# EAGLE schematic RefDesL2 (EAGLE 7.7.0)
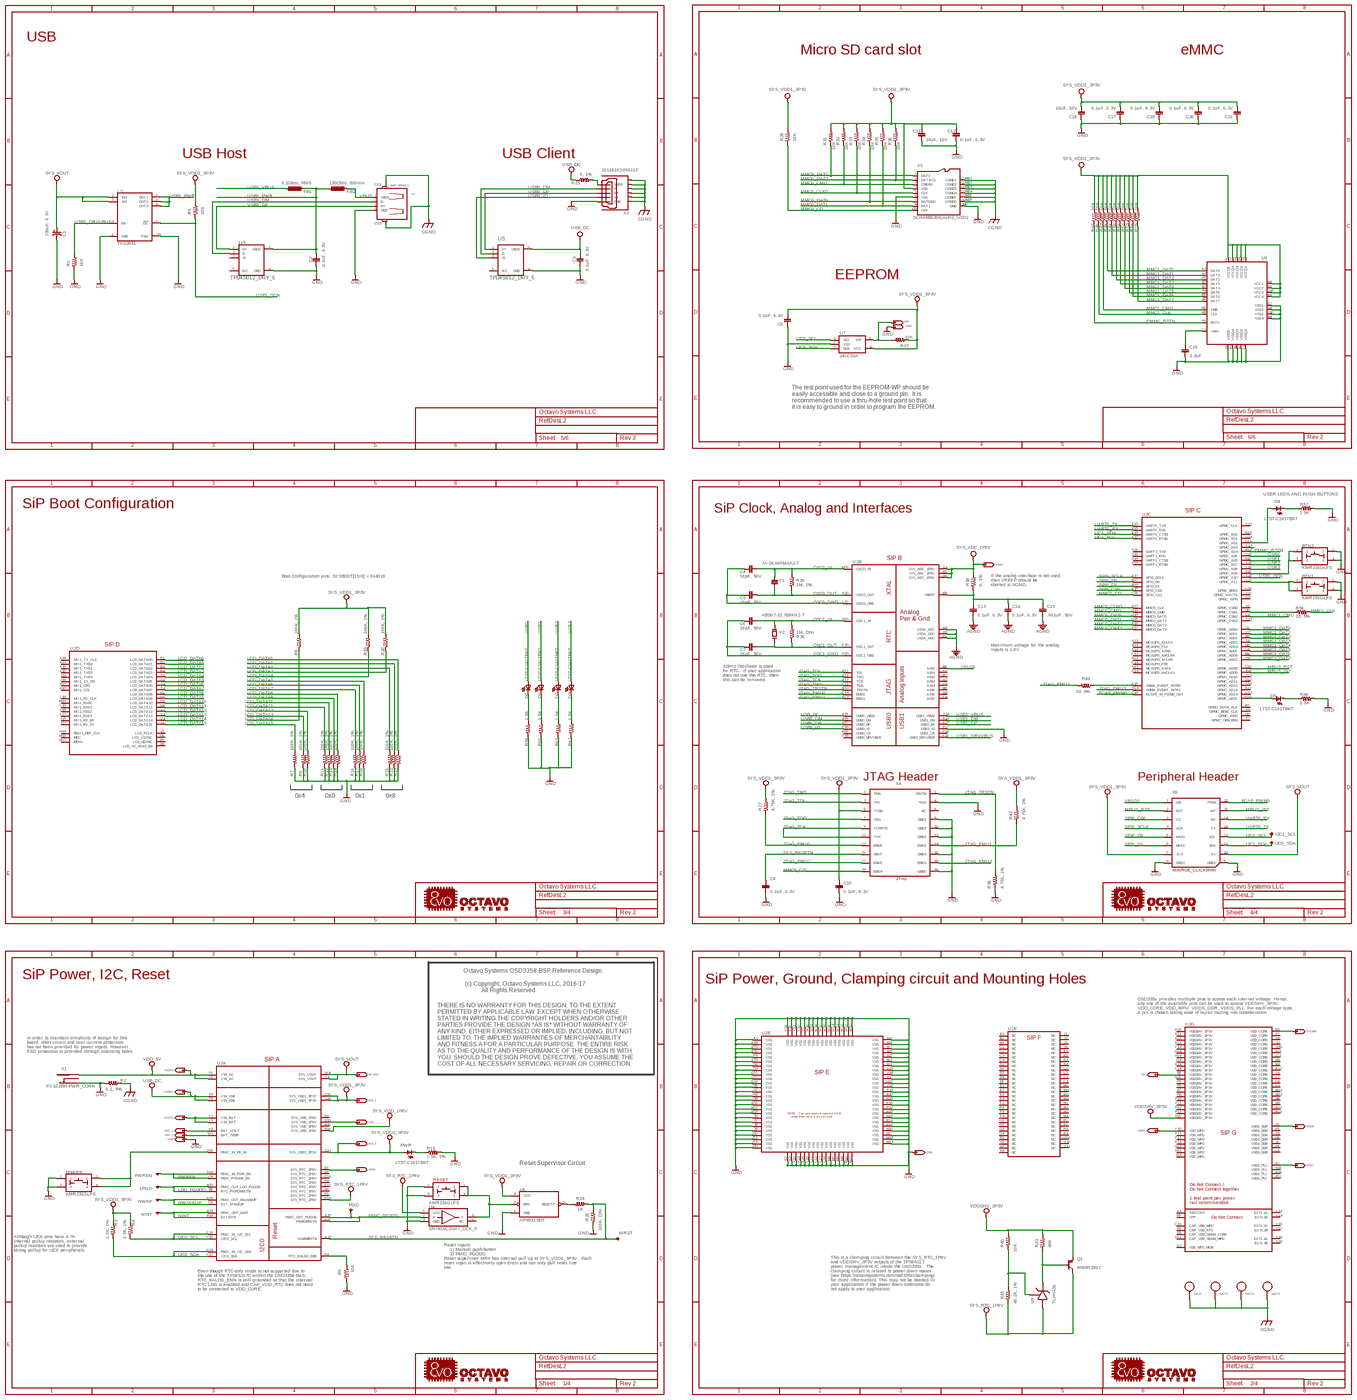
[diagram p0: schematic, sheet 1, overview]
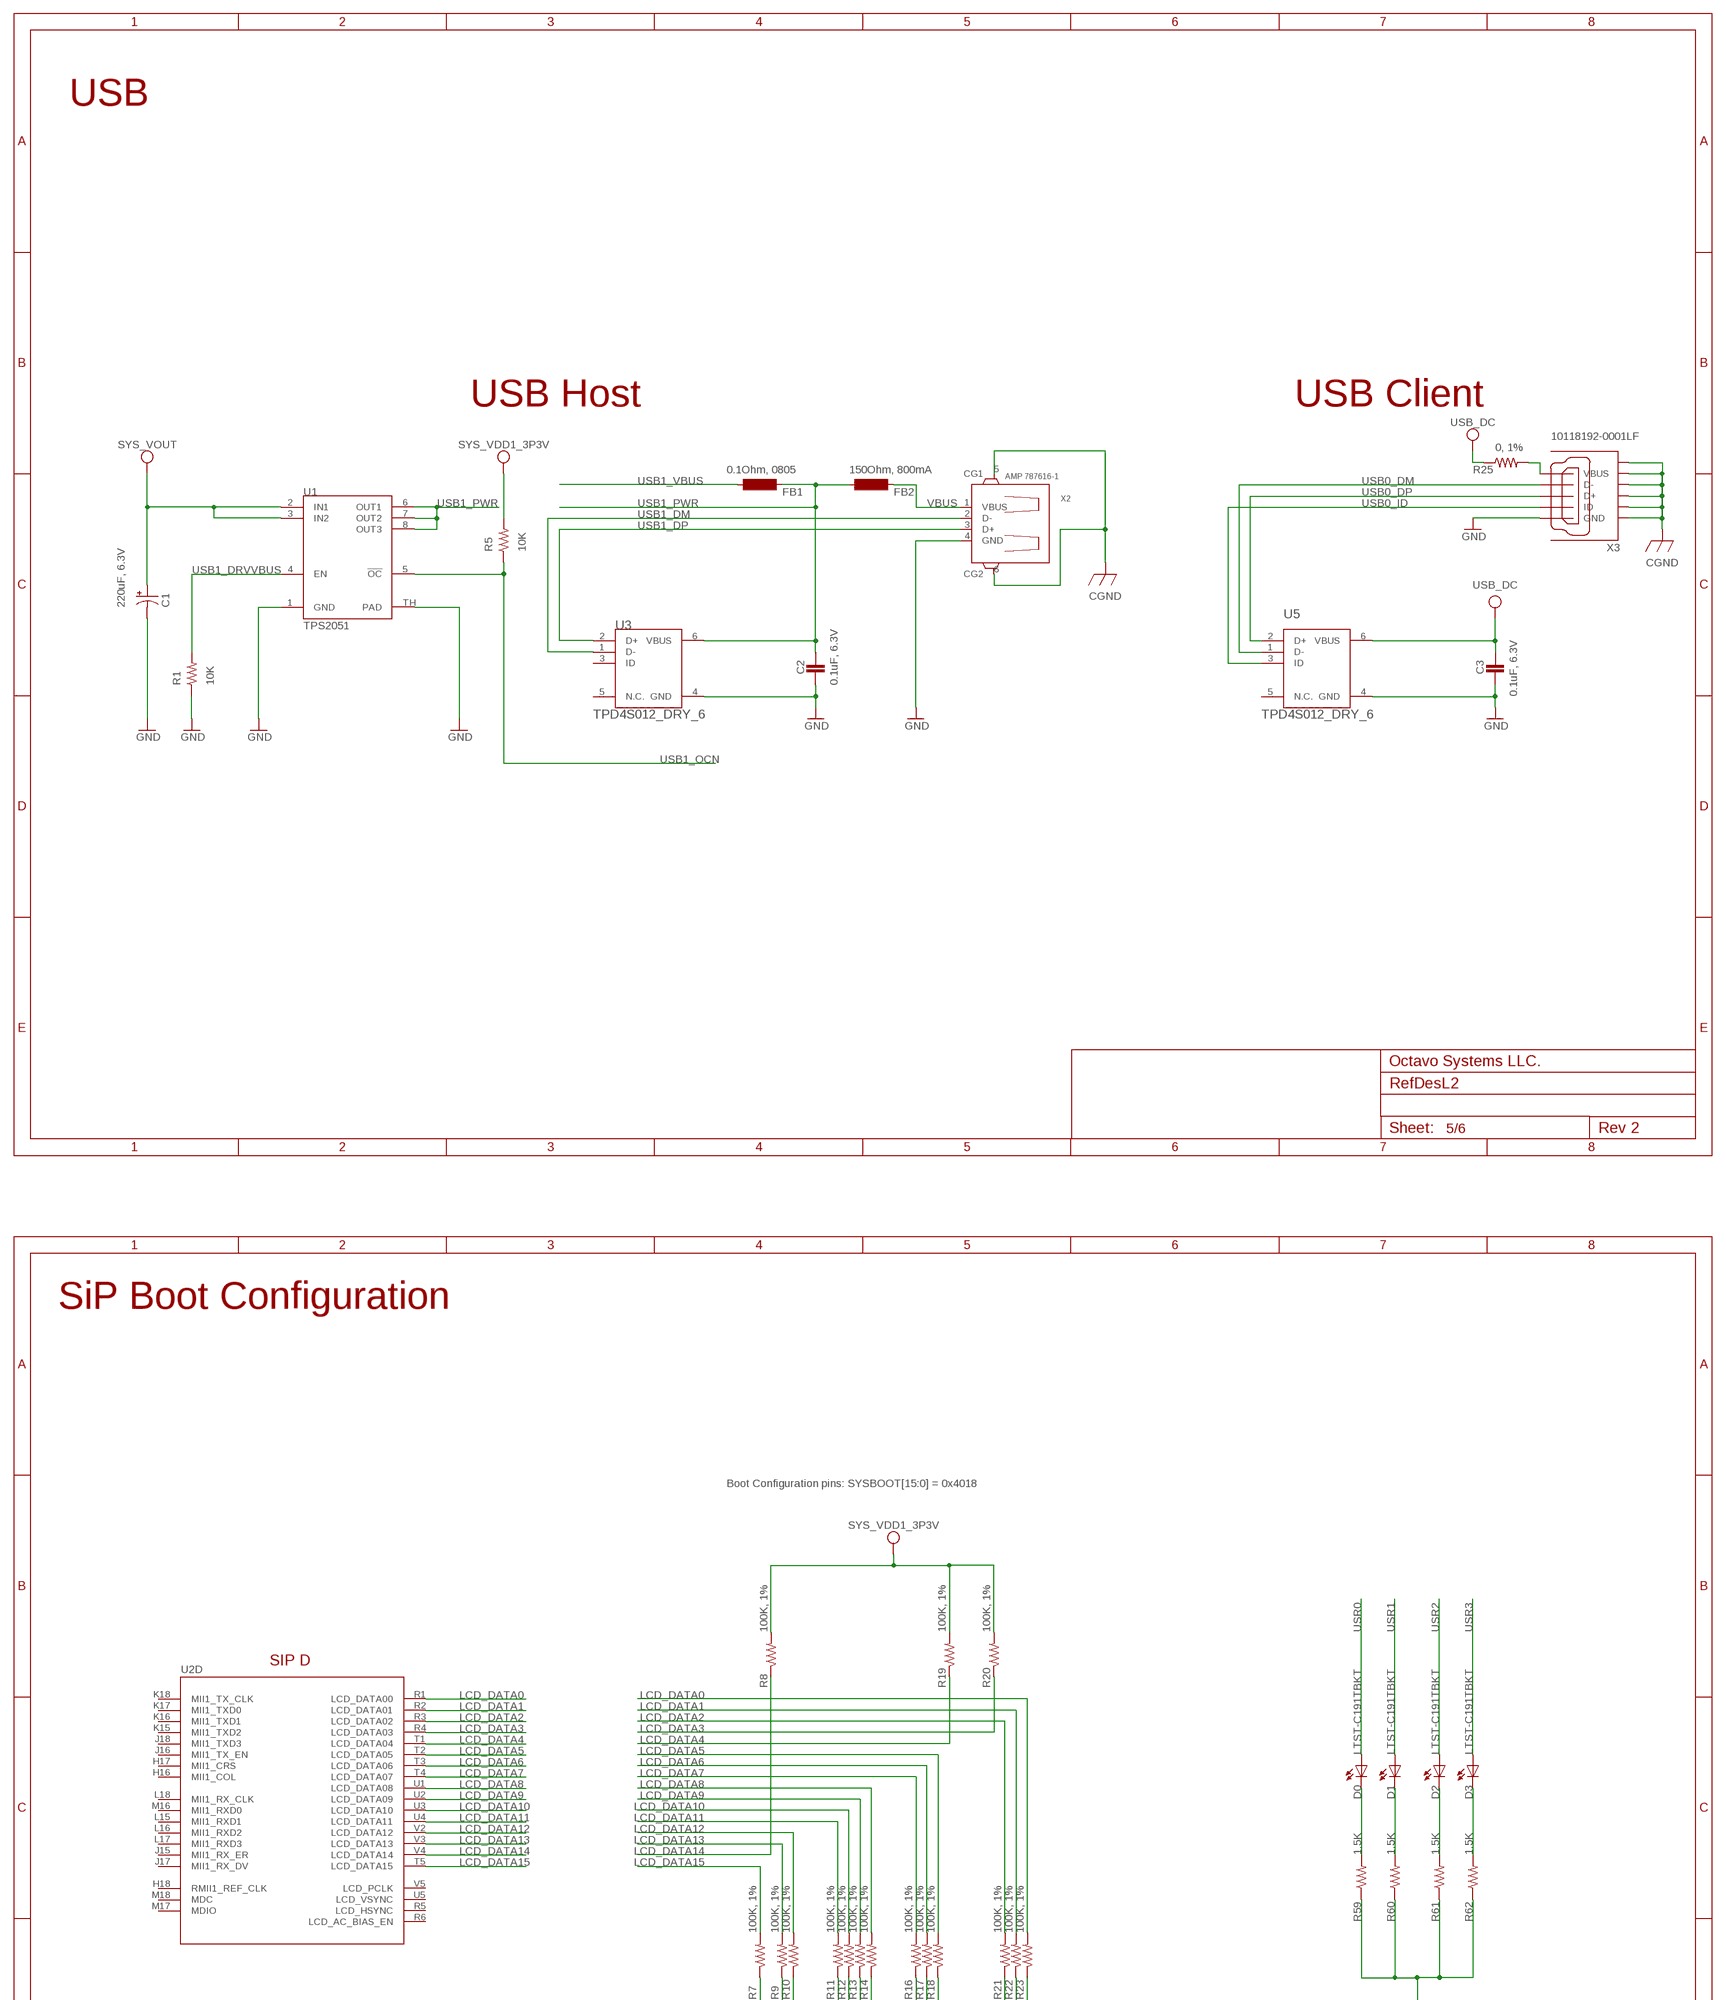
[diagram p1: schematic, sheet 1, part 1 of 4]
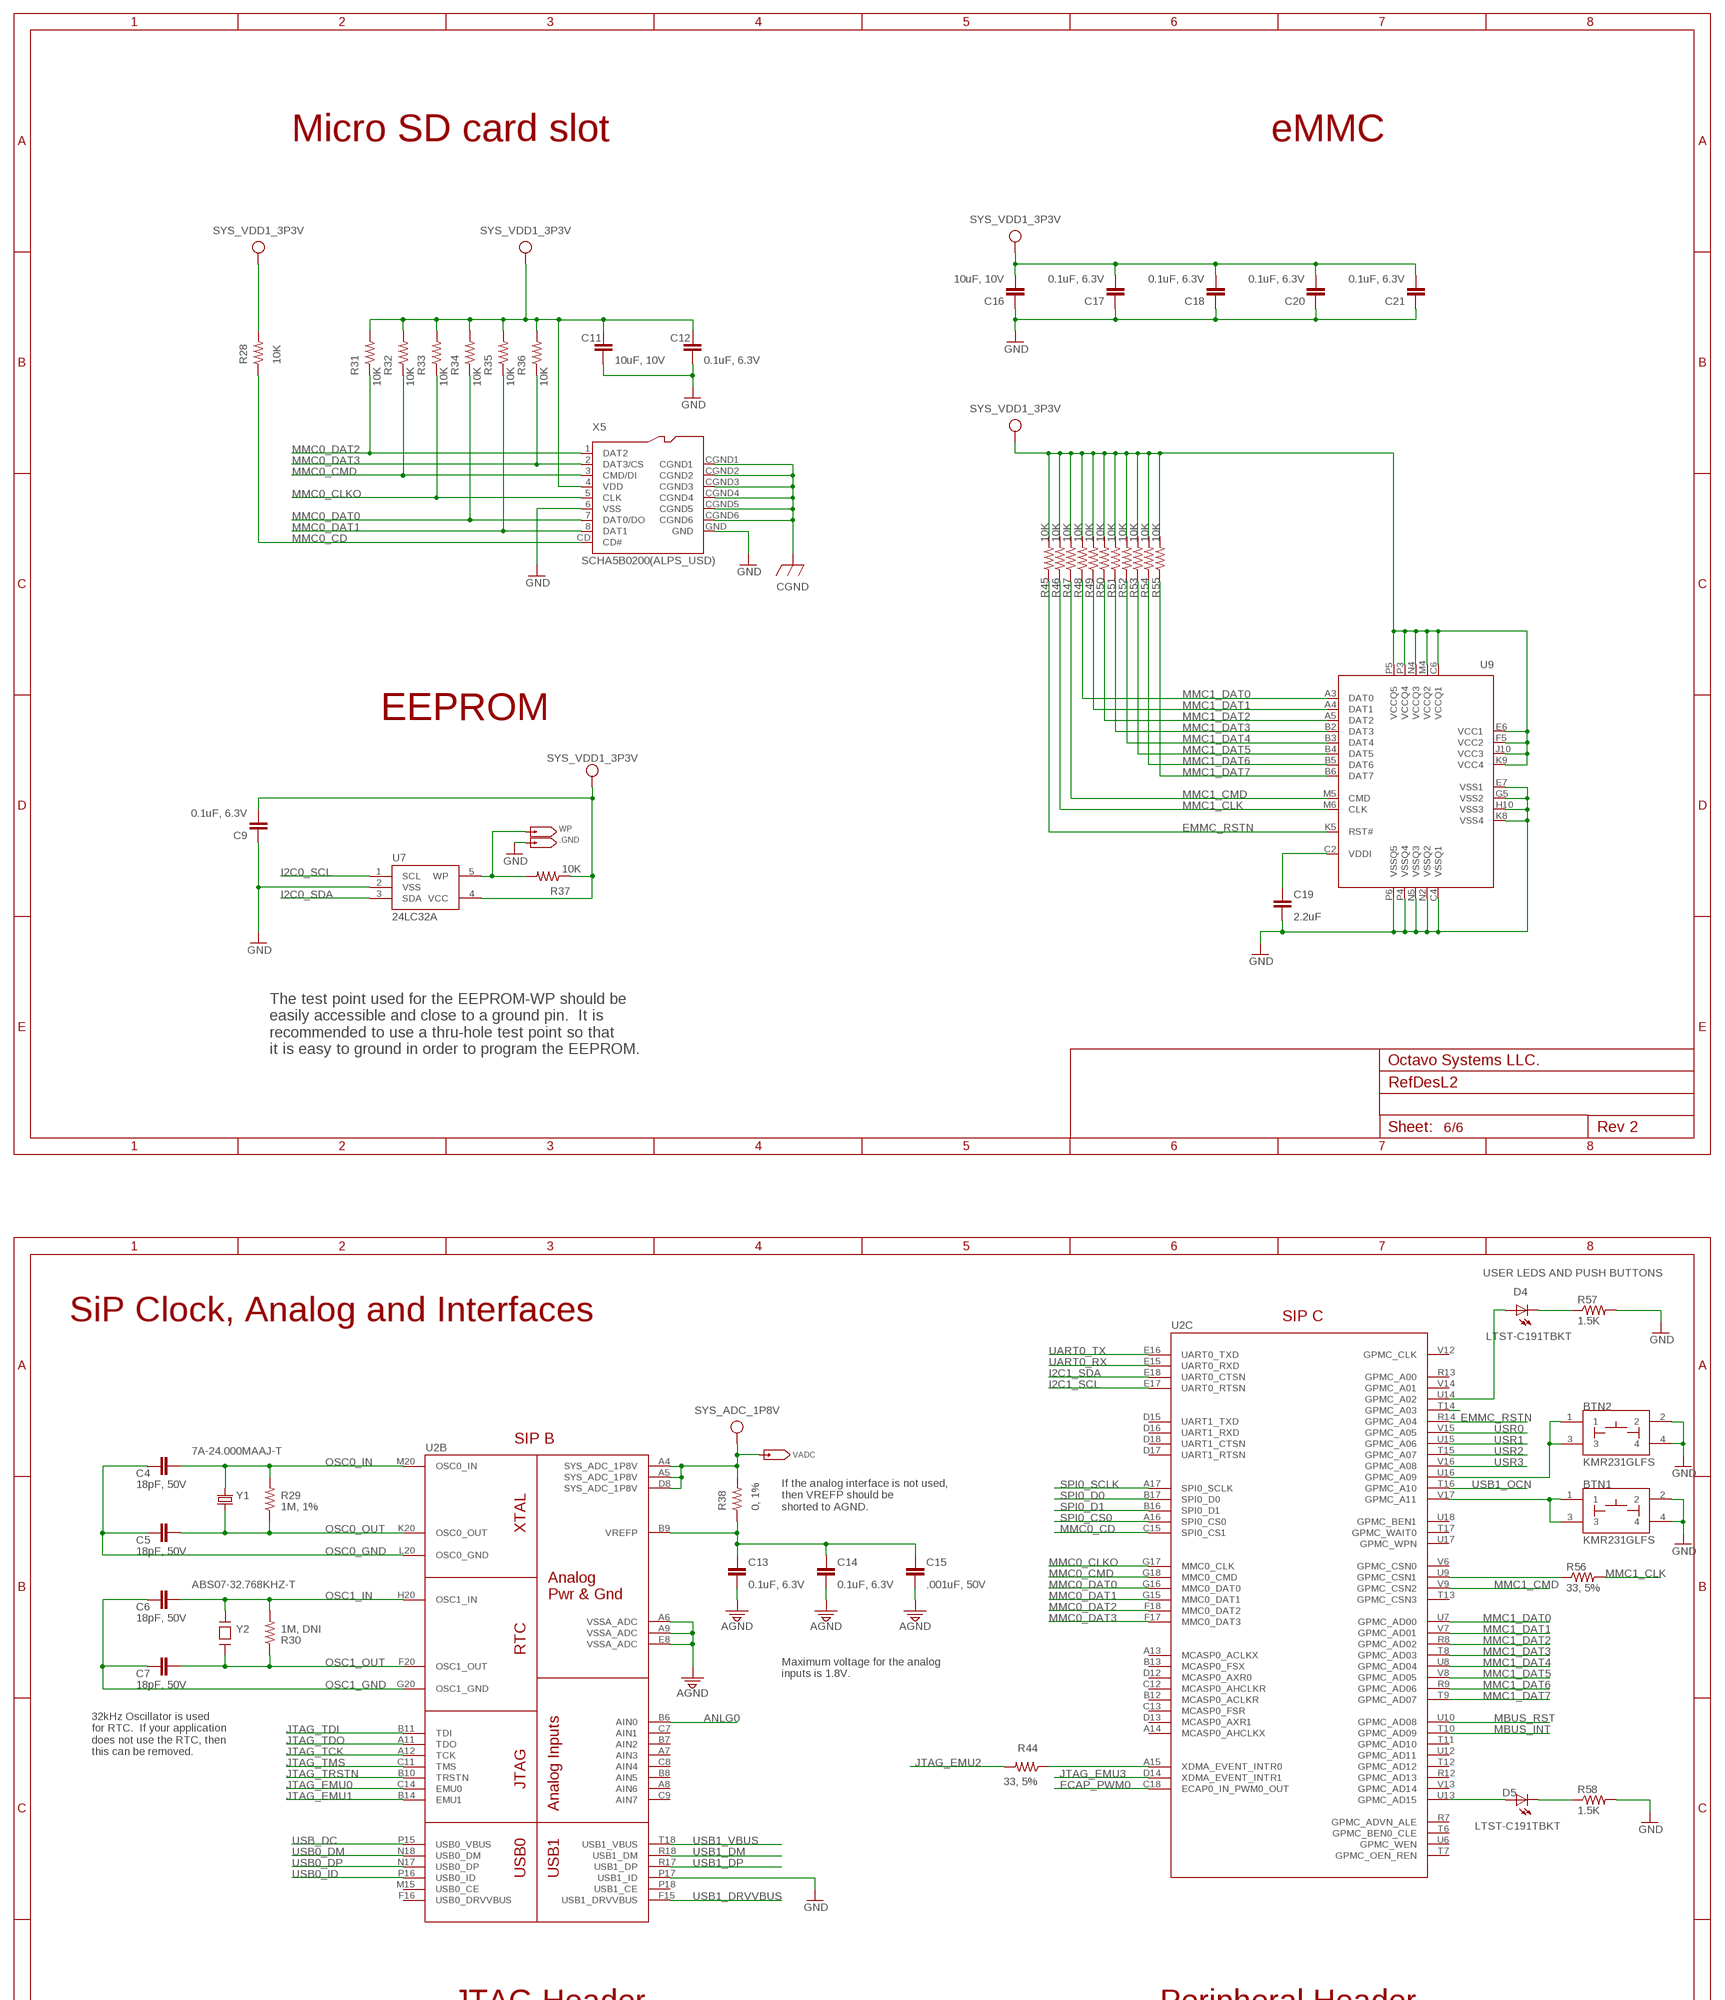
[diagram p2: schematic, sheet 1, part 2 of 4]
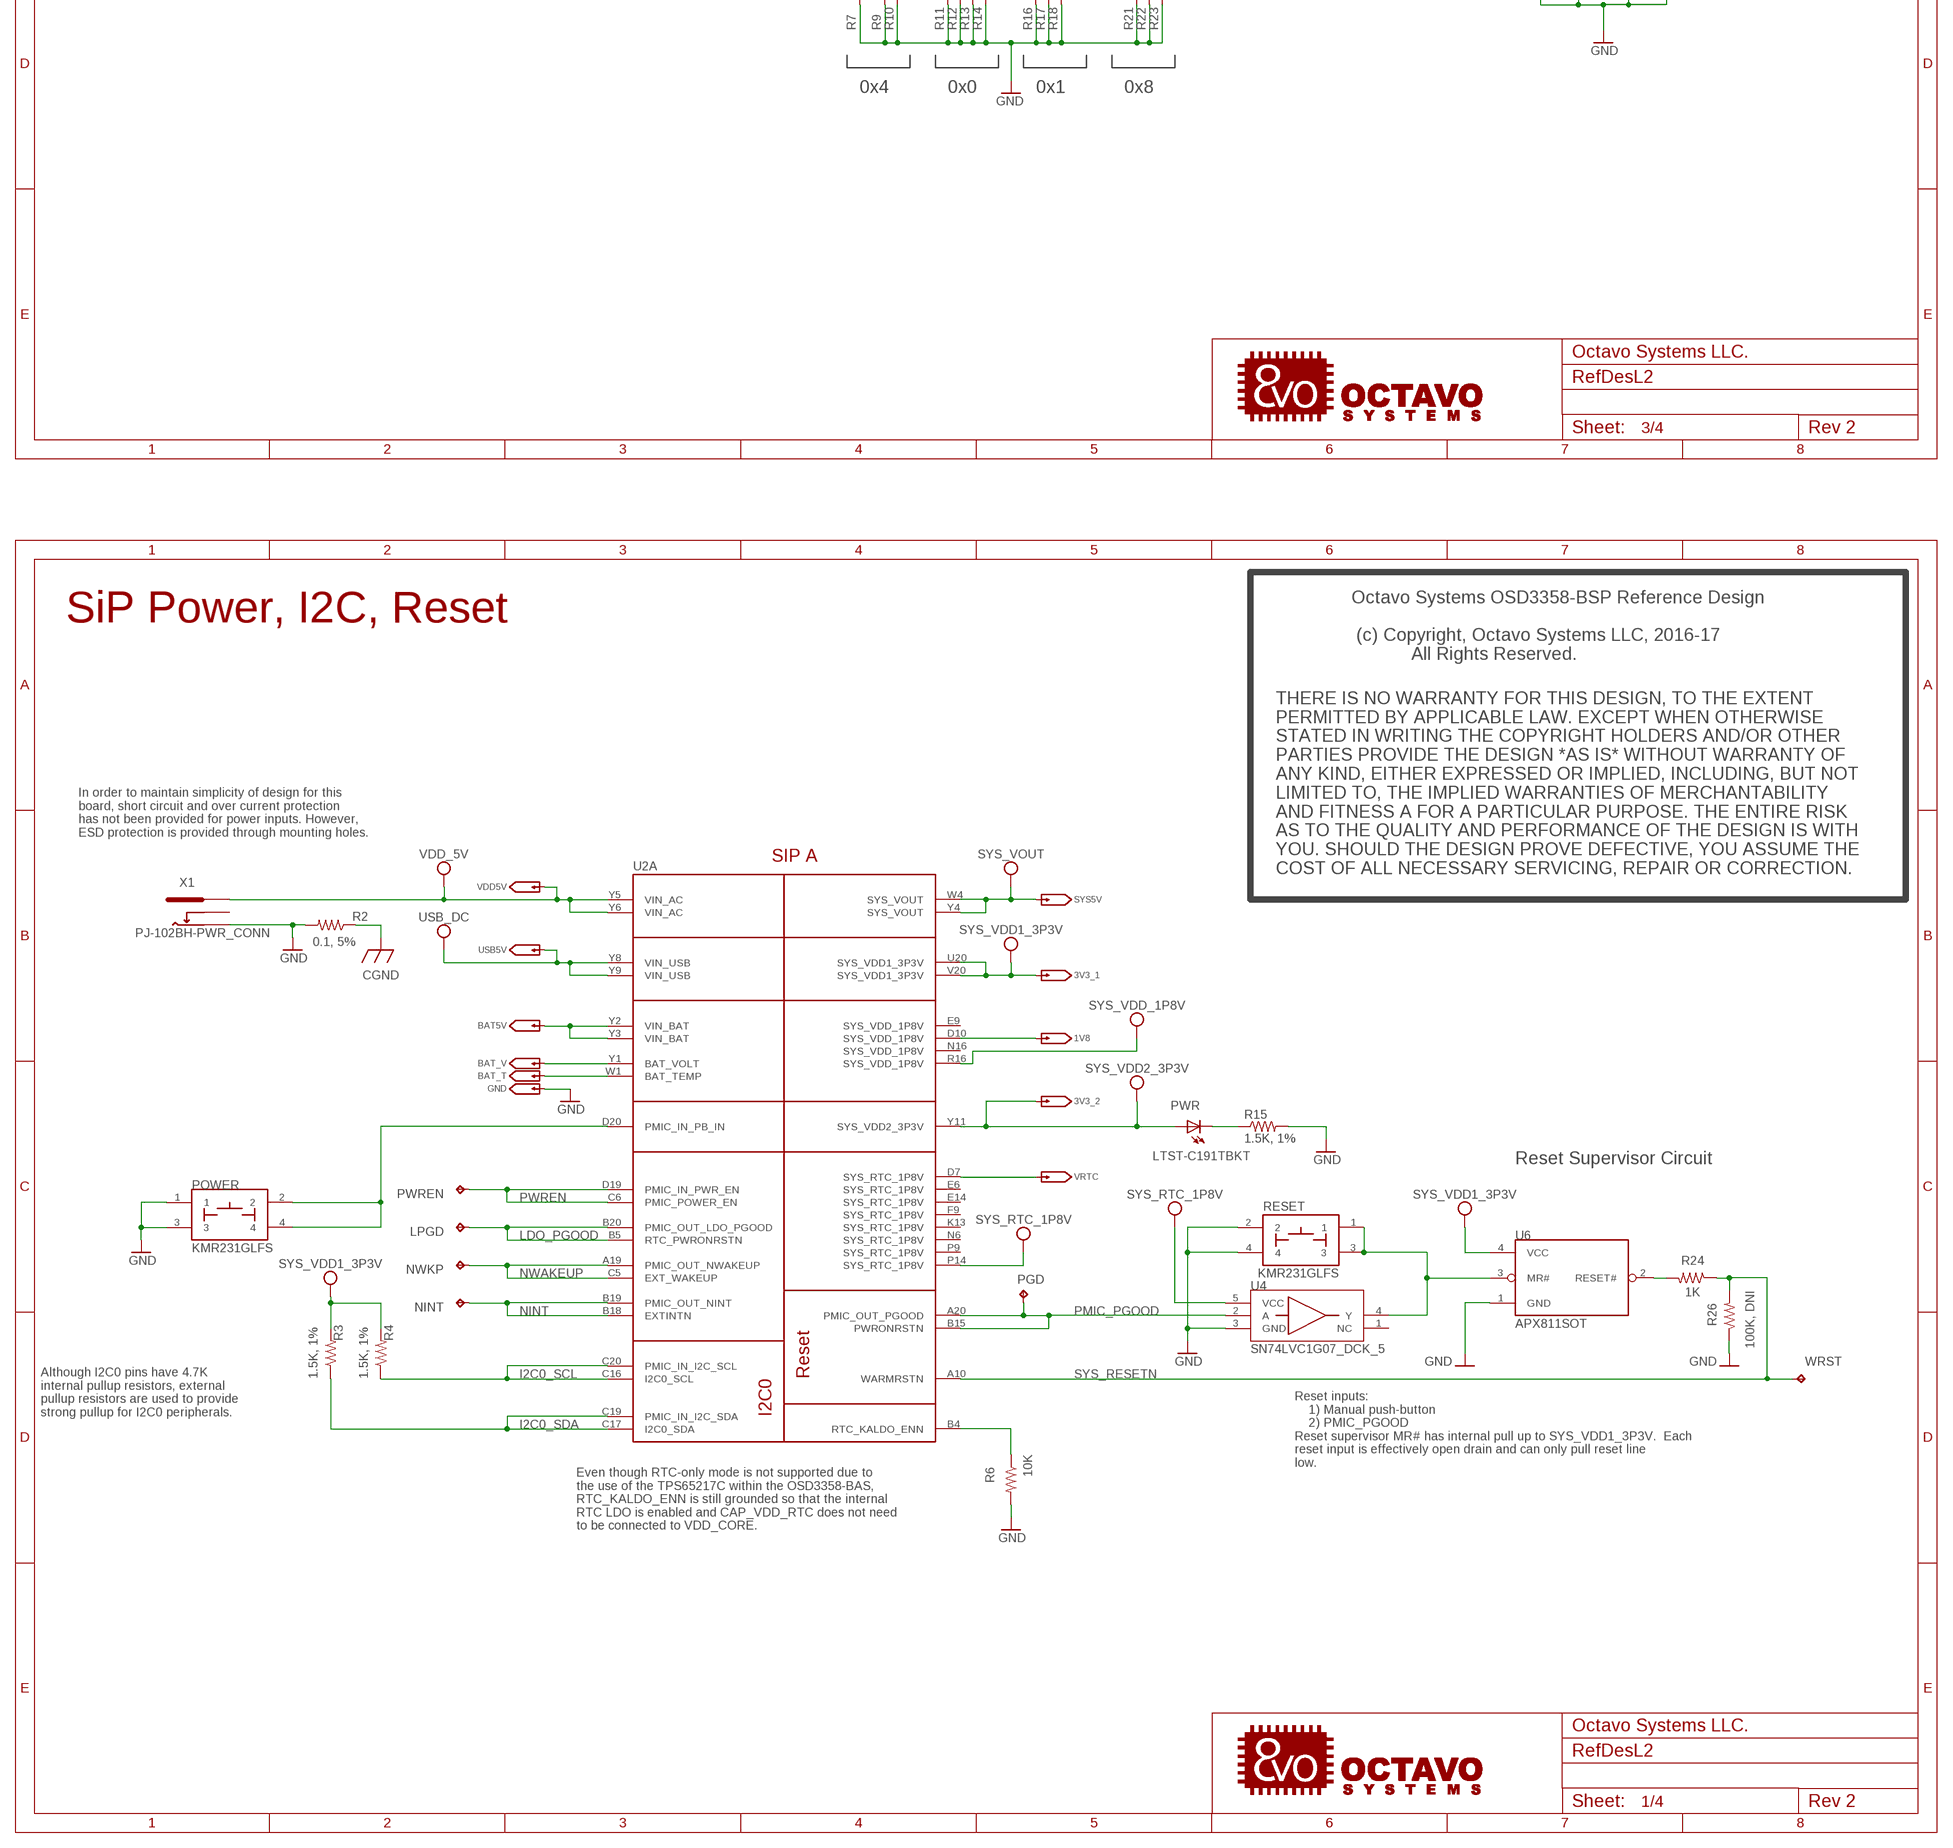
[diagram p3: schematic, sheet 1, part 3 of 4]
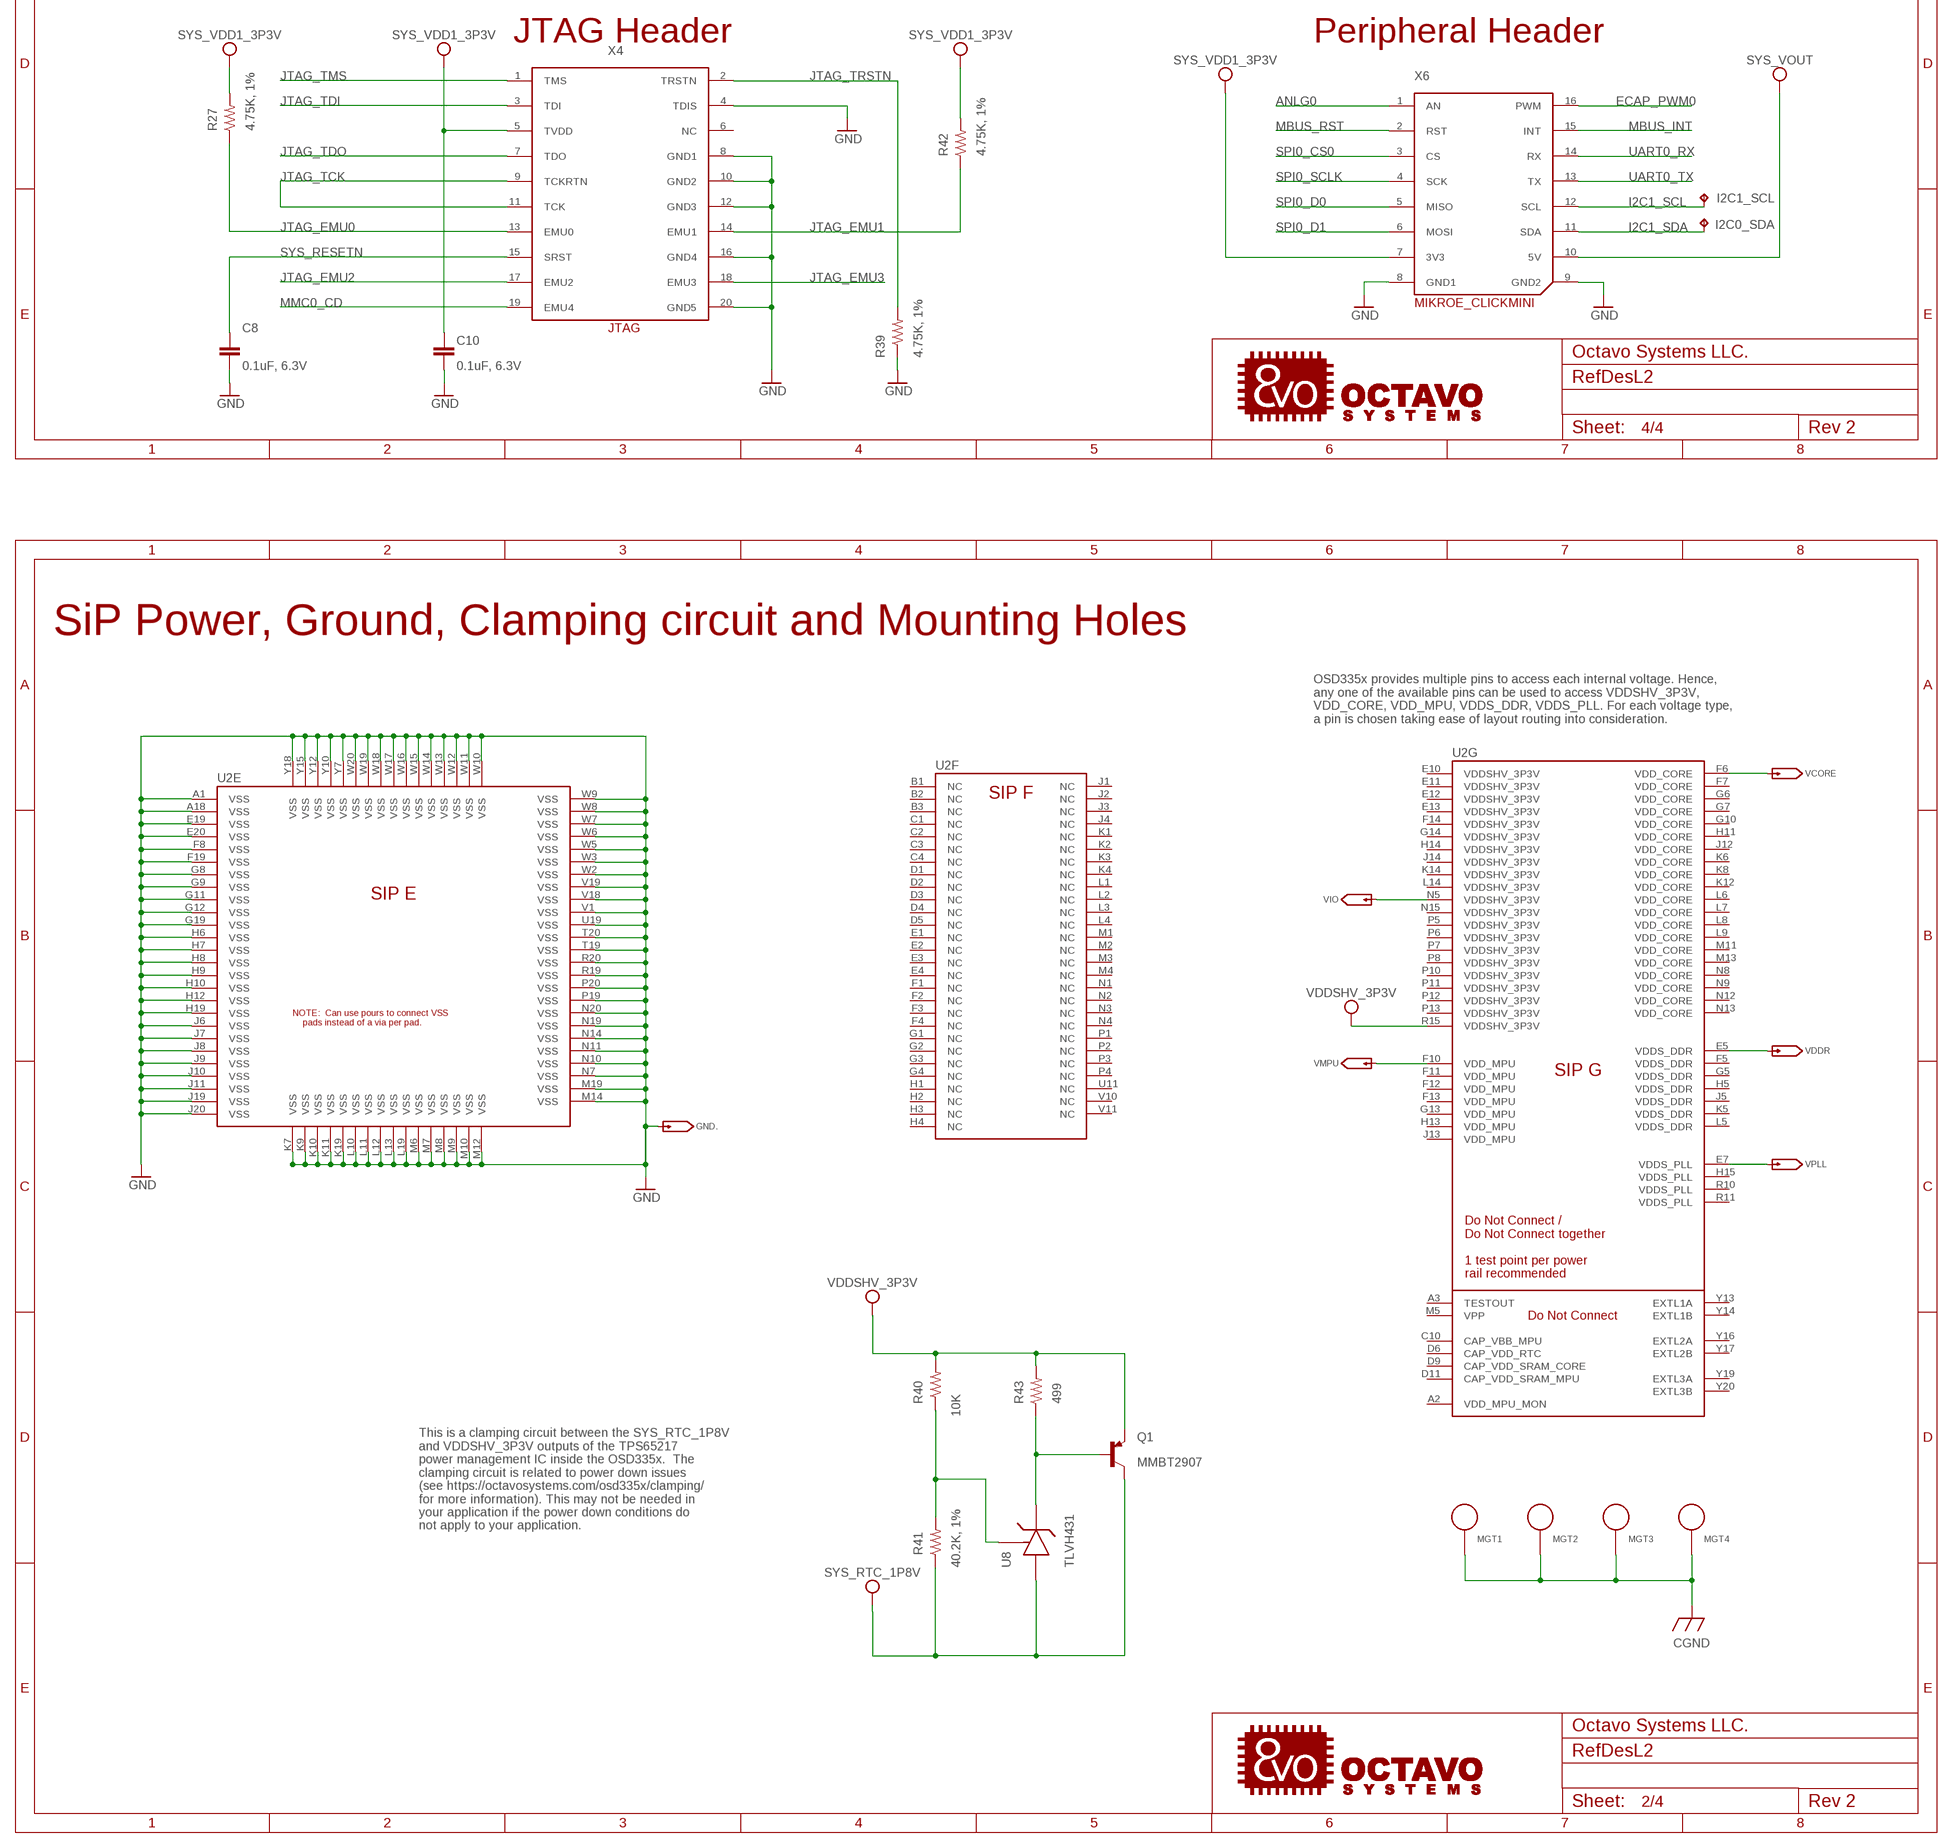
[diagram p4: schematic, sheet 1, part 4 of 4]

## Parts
1V8  TESTPAD/W_HOLE_1X1  [TESTPAD/W_HOLE_1X1]
3V3_1  TESTPAD/W_HOLE_1X1  [TESTPAD/W_HOLE_1X1]
3V3_2  TESTPAD/W_HOLE_1X1  [TESTPAD/W_HOLE_1X1]
.GND  TESTPAD/W_HOLE_1X1  [TESTPAD/W_HOLE_1X1]
BAT5V  TESTPAD/W_HOLE_1X1  [TESTPAD/W_HOLE_1X1]
BAT_T  TESTPAD/W_HOLE_1X1  [TESTPAD/W_HOLE_1X1]
BAT_V  TESTPAD/W_HOLE_1X1  [TESTPAD/W_HOLE_1X1]
BTN1  KMR231GLFS  [SW4SMD_63X161LS]
BTN2  KMR231GLFS  [SW4SMD_63X161LS]
C1  220uF, 6.3V  CPOL-USB/3528-21R  [B/3528-21R]
C2  0.1uF, 6.3V  CC0402  [C0402]
C3  0.1uF, 6.3V  CC0402  [C0402]
C4  18pF, 50V  CC0402  [C0402]
C5  18pF, 50V  CC0402  [C0402]
C6  18pF, 50V  CC0402  [C0402]
C7  18pF, 50V  CC0402  [C0402]
C8  0.1uF, 6.3V  CC0402  [C0402]
C9  0.1uF, 6.3V  CC0402  [C0402]
C10  0.1uF, 6.3V  CC0402  [C0402]
C11  10uF, 10V  CC0805  [C0805]
C12  0.1uF, 6.3V  CC0402  [C0402]
C13  0.1uF, 6.3V  CC0402  [C0402]
C14  0.1uF, 6.3V  CC0402  [C0402]
C15  .001uF, 50V  CC0402  [C0402]
C16  10uF, 10V  CC0805  [C0805]
C17  0.1uF, 6.3V  CC0402  [C0402]
C18  0.1uF, 6.3V  CC0402  [C0402]
C19  2.2uF  CC0402  [C0402]
C20  0.1uF, 6.3V  CC0402  [C0402]
C21  0.1uF, 6.3V  CC0402  [C0402]
D0  LTST-C191TBKT  LTST-C191TBKTLED_EIA-STD  [EIA-STD]
D1  LTST-C191TBKT  LTST-C191TBKTLED_EIA-STD  [EIA-STD]
D2  LTST-C191TBKT  LTST-C191TBKTLED_EIA-STD  [EIA-STD]
D3  LTST-C191TBKT  LTST-C191TBKTLED_EIA-STD  [EIA-STD]
D4  LTST-C191TBKT  LTST-C191TBKTLED_EIA-STD  [EIA-STD]
D5  LTST-C191TBKT  LTST-C191TBKTLED_EIA-STD  [EIA-STD]
FB1  0.1Ohm, 0805  MPZ2012S601AT000FB_0805  [C0805]
FB2  150Ohm, 800mA  MPZ2012S601AT000FB_0805  [C0805]
GND  TESTPAD/W_HOLE_1X1  [TESTPAD/W_HOLE_1X1]
GND.  TESTPAD/W_HOLE_1X1  [TESTPAD/W_HOLE_1X1]
I2C0_SDA  TPTP15R  [TP15R]
I2C1_SCL  TPTP15R  [TP15R]
LPGD  TPTP15R  [TP15R]
MGT1  MOUNTING_HOLE  [MOUNTING_HOLE]
MGT2  MOUNTING_HOLE  [MOUNTING_HOLE]
MGT3  MOUNTING_HOLE  [MOUNTING_HOLE]
MGT4  MOUNTING_HOLE  [MOUNTING_HOLE]
NINT  TPTP15R  [TP15R]
NWKP  TPTP15R  [TP15R]
PGD  TPTP15R  [TP15R]
POWER  KMR231GLFS  [SW4SMD_63X161LS]
PWR  LTST-C191TBKT  LTST-C191TBKTLED_EIA-STD  [EIA-STD]
PWREN  TPTP15R  [TP15R]
Q1  MMBT2907  MMBT2907SMD  [SOT23-BEC]
R1  10K  R-US_R0402  [R0402]
R2  0.1, 5%  R-US_R0805  [R0805]
R3  1.5K, 1%  R-US_R0402  [R0402]
R4  1.5K, 1%  R-US_R0402  [R0402]
R5  10K  R-US_R0402  [R0402]
R6  10K  R-US_R0402  [R0402]
R7  100K, 1%  R-US_R0402  [R0402]
R8  100K, 1%  R-US_R0402  [R0402]
R9  100K, 1%  R-US_R0402  [R0402]
R10  100K, 1%  R-US_R0402  [R0402]
R11  100K, 1%  R-US_R0402  [R0402]
R12  100K, 1%  R-US_R0402  [R0402]
R13  100K, 1%  R-US_R0402  [R0402]
R14  100K, 1%  R-US_R0402  [R0402]
R15  1.5K, 1%  R-US_R0402  [R0402]
R16  100K, 1%  R-US_R0402  [R0402]
R17  100K, 1%  R-US_R0402  [R0402]
R18  100K, 1%  R-US_R0402  [R0402]
R19  100K, 1%  R-US_R0402  [R0402]
R20  100K, 1%  R-US_R0402  [R0402]
R21  100K, 1%  R-US_R0402  [R0402]
R22  100K, 1%  R-US_R0402  [R0402]
R23  100K, 1%  R-US_R0402  [R0402]
R24  1K  R-US_R0402  [R0402]
R25  0, 1%  R-US_R0805  [R0805]
R26  100K, DNI  R-US_R0402  [R0402]
R27  4.75K, 1%  R-US_R0402  [R0402]
R28  10K  R-US_R0402  [R0402]
R29  1M, 1%  R-US_R0402  [R0402]
R30  1M, DNI  R-US_R0402  [R0402]
R31  10K  R-US_R0402  [R0402]
R32  10K  R-US_R0402  [R0402]
R33  10K  R-US_R0402  [R0402]
R34  10K  R-US_R0402  [R0402]
R35  10K  R-US_R0402  [R0402]
R36  10K  R-US_R0402  [R0402]
R37  10K  R-US_R0402  [R0402]
R38  0, 1%  R-US_R0402  [R0402]
R39  4.75K, 1%  R-US_R0402  [R0402]
R40  10K  R-US_R0402  [R0402]
R41  40.2K, 1%  R-US_R0402  [R0402]
R42  4.75K, 1%  R-US_R0402  [R0402]
R43  499  R-US_R0402  [R0402]
R44  33, 5%  R-US_R0402  [R0402]
R45  10K  R-US_R0402  [R0402]
R46  10K  R-US_R0402  [R0402]
R47  10K  R-US_R0402  [R0402]
R48  10K  R-US_R0402  [R0402]
R49  10K  R-US_R0402  [R0402]
R50  10K  R-US_R0402  [R0402]
R51  10K  R-US_R0402  [R0402]
R52  10K  R-US_R0402  [R0402]
R53  10K  R-US_R0402  [R0402]
R54  10K  R-US_R0402  [R0402]
R55  10K  R-US_R0402  [R0402]
R56  33, 5%  R-US_R0402  [R0402]
R57  1.5K  R-US_R0402  [R0402]
R58  1.5K  R-US_R0402  [R0402]
R59  1.5K  R-US_R0402  [R0402]
R60  1.5K  R-US_R0402  [R0402]
R61  1.5K  R-US_R0402  [R0402]
R62  1.5K  R-US_R0402  [R0402]
RESET  KMR231GLFS  [SW4SMD_63X161LS]
SYS5V  TESTPAD/W_HOLE_1X1  [TESTPAD/W_HOLE_1X1]
U1  TPS2051  [S-PDSO-G08]
U2  OSD3358-512M-BAS  [OSD335X-BGA-400]
U3  TPD4S012_DRY_6  [DRY6]
U4  SN74LVC1G07_DCK_5  [DCK5]
U5  TPD4S012_DRY_6  [DRY6]
U6  APX811SOT  [SOT143-R]
U7  24LC32A  [SOT23-5]
U8  TLVH431  [SOT23-3]
U9  EMMC  EMMC04G-S100-B08U  [MICRON_EMMC_153]
USB5V  TESTPAD/W_HOLE_1X1  [TESTPAD/W_HOLE_1X1]
VADC  TESTPAD/W_HOLE_1X1  [TESTPAD/W_HOLE_1X1]
VCORE  TESTPAD/W_HOLE_1X1  [TESTPAD/W_HOLE_1X1]
VDD5V  TESTPAD/W_HOLE_1X1  [TESTPAD/W_HOLE_1X1]
VDDR  TESTPAD/W_HOLE_1X1  [TESTPAD/W_HOLE_1X1]
VIO  TESTPAD/W_HOLE_1X1  [TESTPAD/W_HOLE_1X1]
VMPU  TESTPAD/W_HOLE_1X1  [TESTPAD/W_HOLE_1X1]
VPLL  TESTPAD/W_HOLE_1X1  [TESTPAD/W_HOLE_1X1]
VRTC  TESTPAD/W_HOLE_1X1  [TESTPAD/W_HOLE_1X1]
WP  TESTPAD/W_HOLE_1X1  [TESTPAD/W_HOLE_1X1]
WRST  TPTP15R  [TP15R]
X1  PJ-102BH-PWR_CONN  PJ-102B_POWER_CON  [PJ-102B_POWER_CON]
X2  AMP 787616-1  AMP787616-1  [USB_HOST_HORIZONTAL_W/CHASSIS_GND]
X3  10118192-0001LF  [10118192-0001LF(MICRO-USB-B-AMPHENOL-FCI)]
X4  JTAG  CTI-JTAG  [CTI-JTAG]
X5  SCHA5B0200(ALPS_USD)  [SCHA5B0200]
X6  MIKROE_CLICKMINI  [MIKROE_BUS_MINI]
Y1  7A-24.000MAAJ-T  [CRYSTAL-TXC-7A]
Y2  ABS07-32.768KHZ-T  [CRYSTAL_3.2X1.5]

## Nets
AGND: C13.2 C14.2 C15.2 U2.A6(B:VSSA_ADC) U2.A9(B:VSSA_ADC) U2.E8(B:VSSA_ADC)
ANLG0: U2.B6(B:AIN0) X6.1(AN)
CGND: MGT1.P$1 MGT2.P$1 MGT3.P$1 MGT4.P$1 R2.1 X2.5(CG1) X2.6(CG2) X3.CGND1(SGND1) X3.CGND2(SGND2) X3.CGND3(SGND3) X3.CGND4(SGND4) X3.CGND5(SGND5) X3.CGND6(SGND6) X5.CGND1 X5.CGND2 X5.CGND3 X5.CGND4 X5.CGND5 X5.CGND6
ECAP_PWM0: U2.C18(C:ECAP0_IN_PWM0_OUT) X6.16(PWM)
EMMC_RSTN: R45.1 U2.R14(C:GPMC_A04) U9.K5(RST#)
GND: .GND.P$1(TP) BTN1.2 BTN1.4 BTN2.2 BTN2.4 C1.- C2.2 C3.2 C8.2 C9.1 C10.2 C11.2 C12.2 C16.1 C17.1 C18.1 C19.2 C20.1 C21.1 GND..P$1(TP) GND.P$1(TP) POWER.1 POWER.3 R1.1 R2.2 R6.2 R7.1 R9.1 R10.1 R11.1 R12.1 R13.1 R14.1 R15.2 R16.1 R17.1 R18.1 R21.1 R22.1 R23.1 R26.1 R39.1 R57.2 R58.2 R59.1 R60.1 R61.1 R62.1 RESET.2 RESET.4 U1.1(GND) U1.TH(PAD) U2.A1(E:VSS) U2.A18(E:VSS) U2.E19(E:VSS) U2.E20(E:VSS) U2.F8(E:VSS) U2.F19(E:VSS) U2.G8(E:VSS) U2.G9(E:VSS) U2.G11(E:VSS) U2.G12(E:VSS) U2.G19(E:VSS) U2.H6(E:VSS) U2.H7(E:VSS) U2.H8(E:VSS) U2.H9(E:VSS) U2.H10(E:VSS) U2.H12(E:VSS) U2.H19(E:VSS) U2.J6(E:VSS) U2.J7(E:VSS) U2.J8(E:VSS) U2.J9(E:VSS) U2.J10(E:VSS) U2.J11(E:VSS) U2.J19(E:VSS) U2.J20(E:VSS) U2.K7(E:VSS) U2.K9(E:VSS) U2.K10(E:VSS) U2.K11(E:VSS) U2.K19(E:VSS) U2.L10(E:VSS) U2.L11(E:VSS) U2.L12(E:VSS) U2.L13(E:VSS) U2.L19(E:VSS) U2.M6(E:VSS) U2.M7(E:VSS) U2.M8(E:VSS) U2.M9(E:VSS) U2.M10(E:VSS) U2.M12(E:VSS) U2.M14(E:VSS) U2.M19(E:VSS) U2.N7(E:VSS) U2.N10(E:VSS) U2.N11(E:VSS) U2.N14(E:VSS) U2.N19(E:VSS) U2.N20(E:VSS) U2.P17(B:USB1_ID) U2.P19(E:VSS) U2.P20(E:VSS) U2.R19(E:VSS) U2.R20(E:VSS) U2.T19(E:VSS) U2.T20(E:VSS) U2.U19(E:VSS) U2.V1(E:VSS) U2.V18(E:VSS) U2.V19(E:VSS) U2.W2(E:VSS) U2.W3(E:VSS) U2.W5(E:VSS) U2.W6(E:VSS) U2.W7(E:VSS) U2.W8(E:VSS) U2.W9(E:VSS) U2.W10(E:VSS) U2.W11(E:VSS) U2.W12(E:VSS) U2.W13(E:VSS) U2.W14(E:VSS) U2.W15(E:VSS) U2.W16(E:VSS) U2.W17(E:VSS) U2.W18(E:VSS) U2.W19(E:VSS) U2.W20(E:VSS) U2.Y7(E:VSS) U2.Y10(E:VSS) U2.Y12(E:VSS) U2.Y15(E:VSS) U2.Y18(E:VSS) U3.4(GND) U4.3(GND) U5.4(GND) U6.1(GND) U7.2(VSS) U9.C4(VSSQ1) U9.E7(VSS1) U9.G5(VSS2) U9.H10(VSS3) U9.K8(VSS4) U9.N2(VSSQ2) U9.N5(VSSQ3) U9.P4(VSSQ4) U9.P6(VSSQ5) X1.OUT X2.4(GND) X3.GND X4.4(TDIS) X4.8(GND1) X4.10(GND2) X4.12(GND3) X4.16(GND4) X4.20(GND5) X5.6(VSS) X5.GND X6.8(GND1) X6.9(GND2)
I2C0_SCL: R4.1 U2.C16(A:I2C0_SCL) U2.C20(A:PMIC_IN_I2C_SCL) U7.1(SCL)
I2C0_SDA: R3.1 U2.C17(A:I2C0_SDA) U2.C19(A:PMIC_IN_I2C_SDA) U7.3(SDA)
I2C1_SCL: I2C1_SCL.TP U2.E17(C:UART0_RTSN) X6.12(SCL)
I2C1_SDA: I2C0_SDA.TP U2.E18(C:UART0_CTSN) X6.11(SDA)
JTAG_EMU0: R27.1 U2.C14(B:EMU0) X4.13(EMU0)
JTAG_EMU1: R42.1 U2.B14(B:EMU1) X4.14(EMU1)
JTAG_EMU2: R44.2 X4.17(EMU2)
JTAG_EMU3: U2.D14(C:XDMA_EVENT_INTR1) X4.18(EMU3)
JTAG_TCK: U2.A12(B:TCK) X4.9(TCKRTN) X4.11(TCK)
JTAG_TDI: U2.B11(B:TDI) X4.3(TDI)
JTAG_TDO: U2.A11(B:TDO) X4.7(TDO)
JTAG_TMS: U2.C11(B:TMS) X4.1(TMS)
JTAG_TRSTN: R39.2 U2.B10(B:TRSTN) X4.2(TRSTN)
LCD_DATA0: R23.2 U2.R1(D:LCD_DATA00)
LCD_DATA1: R22.2 U2.R2(D:LCD_DATA01)
LCD_DATA2: R21.2 U2.R3(D:LCD_DATA02)
LCD_DATA3: R20.1 U2.R4(D:LCD_DATA03)
LCD_DATA4: R19.1 U2.T1(D:LCD_DATA04)
LCD_DATA5: R18.2 U2.T2(D:LCD_DATA05)
LCD_DATA6: R17.2 U2.T3(D:LCD_DATA06)
LCD_DATA7: R16.2 U2.T4(D:LCD_DATA07)
LCD_DATA8: R14.2 U2.U1(D:LCD_DATA08)
LCD_DATA9: R13.2 U2.U2(D:LCD_DATA09)
LCD_DATA10: R12.2 U2.U3(D:LCD_DATA10)
LCD_DATA11: R11.2 U2.U4(D:LCD_DATA11)
LCD_DATA12: R10.2 U2.V2(D:LCD_DATA12)
LCD_DATA13: R9.2 U2.V3(D:LCD_DATA13)
LCD_DATA14: R8.1 U2.V4(D:LCD_DATA14)
LCD_DATA15: R7.2 U2.T5(D:LCD_DATA15)
LDO_PGOOD: LPGD.TP U2.B5(A:RTC_PWRONRSTN) U2.B20(A:PMIC_OUT_LDO_PGOOD)
MBUS_INT: U2.T10(C:GPMC_AD09) X6.15(INT)
MBUS_RST: U2.U10(C:GPMC_AD08) X6.2(RST)
MMC0_CD: R28.1 U2.C15(C:SPI0_CS1) X4.19(EMU4) X5.CD(CD#)
MMC0_CLKO: R33.1 U2.G17(C:MMC0_CLK) X5.5(CLK)
MMC0_CMD: R32.1 U2.G18(C:MMC0_CMD) X5.3(CMD/DI)
MMC0_DAT0: R34.1 U2.G16(C:MMC0_DAT0) X5.7(DAT0/DO)
MMC0_DAT1: R35.1 U2.G15(C:MMC0_DAT1) X5.8(DAT1)
MMC0_DAT2: R31.1 U2.F18(C:MMC0_DAT2) X5.1(DAT2)
MMC0_DAT3: R36.1 U2.F17(C:MMC0_DAT3) X5.2(DAT3/CS)
MMC1_CLK: R46.1 R56.2 U9.M6(CLK)
MMC1_CMD: R47.1 U2.V9(C:GPMC_CSN2) U9.M5(CMD)
MMC1_DAT0: R48.1 U2.U7(C:GPMC_AD00) U9.A3(DAT0)
MMC1_DAT1: R49.1 U2.V7(C:GPMC_AD01) U9.A4(DAT1)
MMC1_DAT2: R50.1 U2.R8(C:GPMC_AD02) U9.A5(DAT2)
MMC1_DAT3: R51.1 U2.T8(C:GPMC_AD03) U9.B2(DAT3)
MMC1_DAT4: R52.1 U2.U8(C:GPMC_AD04) U9.B3(DAT4)
MMC1_DAT5: R53.1 U2.V8(C:GPMC_AD05) U9.B4(DAT5)
MMC1_DAT6: R54.1 U2.R9(C:GPMC_AD06) U9.B5(DAT6)
MMC1_DAT7: R55.1 U2.T9(C:GPMC_AD07) U9.B6(DAT7)
N$1: U2.E7(G:VDDS_PLL) VPLL.P$1(TP)
N$2: U2.N5(G:VDDSHV_3P3V) VIO.P$1(TP)
N$3: BAT_V.P$1(TP) U2.Y1(A:BAT_VOLT)
N$4: BAT_T.P$1(TP) U2.W1(A:BAT_TEMP)
N$5: U2.F10(G:VDD_MPU) VMPU.P$1(TP)
N$6: PWR.2(C) R15.1
N$7: U2.F6(G:VDD_CORE) VCORE.P$1(TP)
N$8: U2.E5(G:VDDS_DDR) VDDR.P$1(TP)
N$9: R40.1 R41.2 U8.1(REF)
N$10: Q1.B R43.1 U8.2(CATHODE)
N$11: U2.D7(A:SYS_RTC_1P8V) VRTC.P$1(TP)
N$12: 1V8.P$1(TP) U2.D10(A:SYS_VDD_1P8V)
N$13: R24.2 U6.2(RESET#)
N$14: R56.1 U2.U9(C:GPMC_CSN1)
N$15: R25.2 X3.VBUS
N$16: R44.1 U2.A15(C:XDMA_EVENT_INTR0)
N$17: D0.2(C) R59.2
N$18: D1.2(C) R60.2
N$19: D2.2(C) R61.2
N$20: U2.T14(C:GPMC_A03)
N$21: BTN1.1 BTN1.3 U2.V17(C:GPMC_A11)
N$22: D3.2(C) R62.2
N$24: R6.1 U2.B4(A:RTC_KALDO_ENN)
N$34: D5.2(C) R58.1
N$35: D4.2(C) R57.1
N$36: D5.1(A) U2.U13(C:GPMC_AD15)
N$37: D4.1(A) U2.U14(C:GPMC_A02)
N$38: BTN2.1 BTN2.3 U2.U16(C:GPMC_A09)
N$52: R37.2 U7.5(WP) WP.P$1(TP)
N$81: C19.1 U9.C2(VDDI)
NINT: NINT.TP U2.B18(A:EXTINTN) U2.B19(A:PMIC_OUT_NINT)
NWAKEUP: NWKP.TP U2.A19(A:PMIC_OUT_NWAKEUP) U2.C5(A:EXT_WAKEUP)
OSC0_GND: C4.2 C5.2 U2.L20(B:OSC0_GND)
OSC0_IN: C4.1 R29.2 U2.M20(B:OSC0_IN) Y1.P$2
OSC0_OUT: C5.1 R29.1 U2.K20(B:OSC0_OUT) Y1.P$1
OSC1_GND: C6.2 C7.2 U2.G20(B:OSC1_GND)
OSC1_IN: C6.1 R30.2 U2.H20(B:OSC1_IN) Y2.P$2
OSC1_OUT: C7.1 R30.1 U2.F20(B:OSC1_OUT) Y2.P$1
PMIC_PGOOD: PGD.TP U2.A20(A:PMIC_OUT_PGOOD) U2.B15(A:PWRONRSTN) U4.2(A)
PWR_BUT: POWER.2 POWER.4 U2.D20(A:PMIC_IN_PB_IN)
PWREN: PWREN.TP U2.C6(A:PMIC_POWER_EN) U2.D19(A:PMIC_IN_PWR_EN)
RESET: RESET.1 RESET.3 U4.4(Y) U6.3(MR#)
SPI0_CS0: U2.A16(C:SPI0_CS0) X6.3(CS)
SPI0_D0: U2.B17(C:SPI0_D0) X6.5(MISO)
SPI0_D1: U2.B16(C:SPI0_D1) X6.6(MOSI)
SPI0_SCLK: U2.A17(C:SPI0_SCLK) X6.4(SCK)
SYS_RESETN: C8.1 R24.1 R26.2 U2.A10(A:WARMRSTN) WRST.TP X4.15(SRST)
SYS_RTC_1P8V: Q1.C R41.1 U2.P14(A:SYS_RTC_1P8V) U4.5(VCC) U8.3(ANODE)
SYS_VDD1_3P3V: 3V3_1.P$1(TP) C9.2 C10.1 C11.1 C12.1 C16.2 C17.2 C18.2 C20.2 C21.2 R3.2 R4.2 R5.2 R8.2 R19.2 R20.2 R27.2 R28.2 R31.2 R32.2 R33.2 R34.2 R35.2 R36.2 R37.1 R42.2 R45.2 R46.2 R47.2 R48.2 R49.2 R50.2 R51.2 R52.2 R53.2 R54.2 R55.2 U2.U20(A:SYS_VDD1_3P3V) U2.V20(A:SYS_VDD1_3P3V) U6.4(VCC) U7.4(VCC) U9.C6(VCCQ1) U9.E6(VCC1) U9.F5(VCC2) U9.J10(VCC3) U9.K9(VCC4) U9.M4(VCCQ2) U9.N4(VCCQ3) U9.P3(VCCQ4) U9.P5(VCCQ5) X4.5(TVDD) X5.4(VDD) X6.7(3V3)
SYS_VDD2_3P3V: 3V3_2.P$1(TP) PWR.1(A) U2.Y11(A:SYS_VDD2_3P3V)
SYS_VDD_1P8V: U2.R16(A:SYS_VDD_1P8V)
SYS_VOUT: C1.+ SYS5V.P$1(TP) U1.2(IN1) U1.3(IN2) U2.W4(A:SYS_VOUT) U2.Y4(A:SYS_VOUT) X6.10(5V)
UART0_RX: U2.E15(C:UART0_RXD) X6.14(RX)
UART0_TX: U2.E16(C:UART0_TXD) X6.13(TX)
USB0_DM: U2.N18(B:USB0_DM) U5.1(D-) X3.D-
USB0_DP: U2.N17(B:USB0_DP) U5.2(D+) X3.D+
USB0_ID: U2.P16(B:USB0_ID) U5.3(ID) X3.ID
USB1_DM: U2.R18(B:USB1_DM) U3.1(D-) X2.2(D-)
USB1_DP: U2.R17(B:USB1_DP) U3.2(D+) X2.3(D+)
USB1_DRVVBUS: R1.2 U1.4(EN) U2.F15(B:USB1_DRVVBUS)
USB1_OCN: R5.1 U1.5(!OC) U2.T16(C:GPMC_A10)
USB1_PWR: C2.1 FB1.2 FB2.1 U1.6(OUT1) U1.7(OUT2) U1.8(OUT3) U3.6(VBUS)
USB1_VBUS: FB1.1 U2.T18(B:USB1_VBUS)
USB_DC: C3.1 R25.1 U2.P15(B:USB0_VBUS) U2.Y8(A:VIN_USB) U2.Y9(A:VIN_USB) U5.6(VBUS) USB5V.P$1(TP)
USR0: D0.1(A) U2.V15(C:GPMC_A05)
USR1: D1.1(A) U2.U15(C:GPMC_A06)
USR2: D2.1(A) U2.T15(C:GPMC_A07)
USR3: D3.1(A) U2.V16(C:GPMC_A08)
VBUS: FB2.2 X2.1(VBUS)
VDD_3V3A: Q1.E R40.2 R43.2 U2.R15(G:VDDSHV_3P3V) ; supply symbol labelled VDDSHV_3P3V
VDD_5V: U2.Y5(A:VIN_AC) U2.Y6(A:VIN_AC) VDD5V.P$1(TP) X1.IN
VDD_ADC: R38.2 U2.A4(B:SYS_ADC_1P8V) U2.A5(B:SYS_ADC_1P8V) U2.D8(B:SYS_ADC_1P8V) VADC.P$1(TP) ; supply symbol labelled SYS_ADC_1P8V
VIN_BAT: BAT5V.P$1(TP) U2.Y2(A:VIN_BAT) U2.Y3(A:VIN_BAT)
VREFP_ADC: C13.1 C14.1 C15.1 R38.1 U2.B9(B:VREFP)
Unconnected: U2.A2(G:VDD_MPU_MON) U2.A3(G:TESTOUT) U2.A7(B:AIN3) U2.A8(B:AIN6) U2.A13(C:MCASP0_ACLKX) U2.A14(C:MCASP0_AHCLKX) U2.B1(F:NC) U2.B2(F:NC) U2.B3(F:NC) U2.B7(B:AIN2) U2.B8(B:AIN5) U2.B12(C:MCASP0_ACLKR) U2.B13(C:MCASP0_FSX) U2.C1(F:NC) U2.C2(F:NC) U2.C3(F:NC) U2.C4(F:NC) U2.C7(B:AIN1) U2.C8(B:AIN4) U2.C9(B:AIN7) U2.C10(G:CAP_VBB_MPU) U2.C12(C:MCASP0_AHCLKR) U2.C13(C:MCASP0_FSR) U2.D1(F:NC) U2.D2(F:NC) U2.D3(F:NC) U2.D4(F:NC) U2.D5(F:NC) U2.D6(G:CAP_VDD_RTC) U2.D9(G:CAP_VDD_SRAM_CORE) U2.D11(G:CAP_VDD_SRAM_MPU) U2.D12(C:MCASP0_AXR0) U2.D13(C:MCASP0_AXR1) U2.D15(C:UART1_TXD) U2.D16(C:UART1_RXD) U2.D17(C:UART1_RTSN) U2.D18(C:UART1_CTSN) U2.E1(F:NC) U2.E2(F:NC) U2.E3(F:NC) U2.E4(F:NC) U2.E6(A:SYS_RTC_1P8V) U2.E9(A:SYS_VDD_1P8V) U2.E10(G:VDDSHV_3P3V) U2.E11(G:VDDSHV_3P3V) U2.E12(G:VDDSHV_3P3V) U2.E13(G:VDDSHV_3P3V) U2.E14(A:SYS_RTC_1P8V) U2.F1(F:NC) U2.F2(F:NC) U2.F3(F:NC) U2.F4(F:NC) U2.F5(G:VDDS_DDR) U2.F7(G:VDD_CORE) U2.F9(A:SYS_RTC_1P8V) U2.F11(G:VDD_MPU) U2.F12(G:VDD_MPU) U2.F13(G:VDD_MPU) U2.F14(G:VDDSHV_3P3V) U2.F16(B:USB0_DRVVBUS) U2.G1(F:NC) U2.G2(F:NC) U2.G3(F:NC) U2.G4(F:NC) U2.G5(G:VDDS_DDR) U2.G6(G:VDD_CORE) U2.G7(G:VDD_CORE) U2.G10(G:VDD_CORE) U2.G13(G:VDD_MPU) U2.G14(G:VDDSHV_3P3V) U2.H1(F:NC) U2.H2(F:NC) U2.H3(F:NC) U2.H4(F:NC) U2.H5(G:VDDS_DDR) U2.H11(G:VDD_CORE) U2.H13(G:VDD_MPU) U2.H14(G:VDDSHV_3P3V) U2.H15(G:VDDS_PLL) U2.H16(D:MII1_COL) U2.H17(D:MII1_CRS) U2.H18(D:RMII1_REF_CLK) U2.J1(F:NC) U2.J2(F:NC) U2.J3(F:NC) U2.J4(F:NC) U2.J5(G:VDDS_DDR) U2.J12(G:VDD_CORE) U2.J13(G:VDD_MPU) U2.J14(G:VDDSHV_3P3V) U2.J15(D:MII1_RX_ER) U2.J16(D:MII1_TX_EN) U2.J17(D:MII1_RX_DV) U2.J18(D:MII1_TXD3) U2.K1(F:NC) U2.K2(F:NC) U2.K3(F:NC) U2.K4(F:NC) U2.K5(G:VDDS_DDR) U2.K6(G:VDD_CORE) U2.K8(G:VDD_CORE) U2.K12(G:VDD_CORE) U2.K13(A:SYS_RTC_1P8V) U2.K14(G:VDDSHV_3P3V) U2.K15(D:MII1_TXD2) U2.K16(D:MII1_TXD1) U2.K17(D:MII1_TXD0) U2.K18(D:MII1_TX_CLK) U2.L1(F:NC) U2.L2(F:NC) U2.L3(F:NC) U2.L4(F:NC) U2.L5(G:VDDS_DDR) U2.L6(G:VDD_CORE) U2.L7(G:VDD_CORE) U2.L8(G:VDD_CORE) U2.L9(G:VDD_CORE) U2.L14(G:VDDSHV_3P3V) U2.L15(D:MII1_RXD1) U2.L16(D:MII1_RXD2) U2.L17(D:MII1_RXD3) U2.L18(D:MII1_RX_CLK) U2.M1(F:NC) U2.M2(F:NC) U2.M3(F:NC) U2.M4(F:NC) U2.M5(G:VPP) U2.M11(G:VDD_CORE) U2.M13(G:VDD_CORE) U2.M15(B:USB0_CE) U2.M16(D:MII1_RXD0) U2.M17(D:MDIO) U2.M18(D:MDC) U2.N1(F:NC) U2.N2(F:NC) U2.N3(F:NC) U2.N4(F:NC) U2.N6(A:SYS_RTC_1P8V) U2.N8(G:VDD_CORE) U2.N9(G:VDD_CORE) U2.N12(G:VDD_CORE) U2.N13(G:VDD_CORE) U2.N15(G:VDDSHV_3P3V) U2.N16(A:SYS_VDD_1P8V) U2.P1(F:NC) U2.P2(F:NC) U2.P3(F:NC) U2.P4(F:NC) U2.P5(G:VDDSHV_3P3V) U2.P6(G:VDDSHV_3P3V) U2.P7(G:VDDSHV_3P3V) U2.P8(G:VDDSHV_3P3V) U2.P9(A:SYS_RTC_1P8V) U2.P10(G:VDDSHV_3P3V) U2.P11(G:VDDSHV_3P3V) U2.P12(G:VDDSHV_3P3V) U2.P13(G:VDDSHV_3P3V) U2.P18(B:USB1_CE) U2.R5(D:LCD_HSYNC) U2.R6(D:LCD_AC_BIAS_EN) U2.R7(C:GPMC_ADVN_ALE) U2.R10(G:VDDS_PLL) U2.R11(G:VDDS_PLL) U2.R12(C:GPMC_AD13) U2.R13(C:GPMC_A00) U2.T6(C:GPMC_BEN0_CLE) U2.T7(C:GPMC_OEN_REN) U2.T11(C:GPMC_AD10) U2.T12(C:GPMC_AD12) U2.T13(C:GPMC_CSN3) U2.T17(C:GPMC_WAIT0) U2.U5(D:LCD_VSYNC) U2.U6(C:GPMC_WEN) U2.U11(F:NC) U2.U12(C:GPMC_AD11) U2.U17(C:GPMC_WPN) U2.U18(C:GPMC_BEN1) U2.V5(D:LCD_PCLK) U2.V6(C:GPMC_CSN0) U2.V10(F:NC) U2.V11(F:NC) U2.V12(C:GPMC_CLK) U2.V13(C:GPMC_AD14) U2.V14(C:GPMC_A01) U2.Y13(G:EXTL1A) U2.Y14(G:EXTL1B) U2.Y16(G:EXTL2A) U2.Y17(G:EXTL2B) U2.Y19(G:EXTL3A) U2.Y20(G:EXTL3B) U3.3(ID) U3.5(N.C.) U4.1(NC) U5.5(N.C.) X1.OUT_CON X4.6(NC)

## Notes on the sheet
- USB
- Micro SD card slot | eMMC
- USB Host | USB Client
- EEPROM
- The test point used for the EEPROM-WP should be
  easily accessible and close to a ground pin.  It is
  recommended to use a thru-hole test point so that
  it is easy to ground in order to program the EEPROM.
- 5/6 | 6/6
- USER LEDS AND PUSH BUTTONS
- SiP Boot Configuration
- SiP Clock, Analog and Interfaces
- Boot Configuration pins: SYSBOOT[15:0] = 0x4018
- If the analog interface is not used,
  then VREFP should be
  shorted to AGND.
- Maximum voltage for the analog
  inputs is 1.8V.
- 32kHz Oscillator is used
  for RTC.  If your application
  does not use the RTC, then
  this can be removed.
- JTAG Header | Peripheral Header
- 0x4 | 0x0 | 0x1 | 0x8
- 3/4 | 4/4
- SiP Power, I2C, Reset | SiP Power, Ground, Clamping circuit and Mounting Holes
- Octavo Systems OSD3358-BSP Reference Design
  
   (c) Copyright, Octavo Systems LLC, 2016-17
              All Rights Reserved.
- OSD335x provides multiple pins to access each internal voltage. Hence,
  any one of the available pins can be used to access VDDSHV_3P3V,
  VDD_CORE, VDD_MPU, VDDS_DDR, VDDS_PLL. For each voltage type,
  a pin is chosen taking ease of layout routing into consideration.
- In order to maintain simplicity of design for this
  board, short circuit and over current protection
  has not been provided for power inputs. However,
  ESD protection is provided through mounting holes.
- THERE IS NO WARRANTY FOR THIS DESIGN, TO THE EXTENT
  PERMITTED BY APPLICABLE LAW. EXCEPT WHEN OTHERWISE
  STATED IN WRITING THE COPYRIGHT HOLDERS AND/OR OTHER
  PARTIES PROVIDE THE DESIGN *AS IS* WITHOUT WARRANTY OF
  ANY KIND, EITHER EXPRESSED OR IMPLIED, INCLUDING, BUT NOT
  LIMITED TO, THE IMPLIED WARRANTIES OF MERCHANTABILITY
  AND FITNESS A FOR A PARTICULAR PURPOSE. THE ENTIRE RISK
  AS TO THE QUALITY AND PERFORMANCE OF THE DESIGN IS WITH
  YOU. SHOULD THE DESIGN PROVE DEFECTIVE, YOU ASSUME THE
  COST OF ALL NECESSARY SERVICING, REPAIR OR CORRECTION.
- Reset Supervisor Circuit
- Although I2C0 pins have 4.7K
  internal pullup resistors, external
  pullup resistors are used to provide
  strong pullup for I2C0 peripherals.
- Reset inputs:
      1) Manual push-button
      2) PMIC_PGOOD
  Reset supervisor MR# has internal pull up to SYS_VDD1_3P3V.  Each
  reset input is effectively open drain and can only pull reset line
  low.
- Even though RTC-only mode is not supported due to
  the use of the TPS65217C within the OSD3358-BAS,
  RTC_KALDO_ENN is still grounded so that the internal
  RTC LDO is enabled and CAP_VDD_RTC does not need
  to be connected to VDD_CORE.
- This is a clamping circuit between the SYS_RTC_1P8V
  and VDDSHV_3P3V outputs of the TPS65217
  power management IC inside the OSD335x.  The
  clamping circuit is related to power down issues
  (see https://octavosystems.com/osd335x/clamping/
  for more information). This may not be needed in
  your application if the power down conditions do
  not apply to your application.
- 1/4 | 2/4

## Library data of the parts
1V8 3V3_1 3V3_2 .GND BAT5V BAT_T BAT_V GND GND. SYS5V USB5V VADC VCORE VDD5V VDDR VIO VMPU VPLL VRTC WP = OSD3358_BAS_RefDesignParts_L2:TESTPAD/W_HOLE_1X1: Test point (Through hole)
BTN1 BTN2 POWER RESET = OSD3358_BAS_RefDesignParts_L2:KMR231GLFS
C1 = OSD3358_BAS_RefDesignParts_L2:CPOL-US: POLARIZED CAPACITOR, American symbol
C2-C21 = OSD3358_BAS_RefDesignParts_L2:C: Capacitor SMD.
D0 D1-D5 PWR = OSD3358_BAS_RefDesignParts_L2:LTST-C191TBKT: PointLED® Enhanced Thinfilm LED TOP & BOTTOM mount
FB1 FB2 = OSD3358_BAS_RefDesignParts_L2:MPZ2012S601AT000: INDUCTOR
I2C0_SDA I2C1_SCL LPGD NINT NWKP PGD PWREN WRST = OSD3358_BAS_RefDesignParts_L2:TP: Test pad
MGT1-MGT4 = OSD3358_BAS_RefDesignParts_L2:MOUNTING_HOLE: Chassis Mounting Hole w/GND connection ability
Q1 = OSD3358_BAS_RefDesignParts_L2:MMBT2907*: PNP Transistror
R1-R62 = OSD3358_BAS_RefDesignParts_L2:R-US_: RESISTOR, American symbol
U1 = OSD3358_BAS_RefDesignParts_L2:TPS2051
U2 = OSD3358_BAS_RefDesignParts_L2:OSD3358-512M-BAS: Octavo Systems LLC OSD335x Family SiP: 27mm x 27mm, 1.27mm pitch 400 pin BGA contains AM3358, 512MB DDR3, TPS65217, TL5209 and passives. Commerical Temperature: 0C to 85C.
U3 U5 = OSD3358_BAS_RefDesignParts_L2:TPD4S012_DRY_6; DATASHEETURL: http://www.ti.com/lit/gpn/TPD4S012; FAMILY_NAME: ESD Solution; GENERIC_PART_NUMBER: TPD4S012; INDUSTRY_STD_PKG_TYPE: SON; MANUFACTURER: Texas Instruments; MANUFACTURER_PART_NUMBER: tpd4s012_dry_6; PACKAGE_DESIGNATOR: DRY; PIN_COUNT: 6; VENDOR: Texas Instruments
U4 = OSD3358_BAS_RefDesignParts_L2:SN74LVC1G07_DCK_5; DATASHEETURL: http://www.ti.com/lit/gpn/SN74LVC1G07; FAMILY_NAME: LL BUFFER AND DRIVER WITH OPEN-DRAIN OUTPUT; GENERIC_PART_NUMBER: SN74LVC1G07; INDUSTRY_STD_PKG_TYPE: SC70; MANUFACTURER: Texas Instruments; MANUFACTURER_PART_NUMBER: sn74lvc1g07_dck_5; PACKAGE_DESIGNATOR: DCK; PIN_COUNT: 5; VENDOR: Texas Instruments
U6 = OSD3358_BAS_RefDesignParts_L2:APX811: Diodes APX811/812 4-pin Microprocessor Supervisor with Manual Reset. Datasheet Footprint Digikey Footprint compatible devices: STM811 Digikey STM6315 Digikey ADM811
U7 = OSD3358_BAS_RefDesignParts_L2:24LC32A: 32K i2c Serial EEPROM
U8 = OSD3358_BAS_RefDesignParts_L2:TLVH431
U9 = OSD3358_BAS_RefDesignParts_L2:EMMC04G-S100-B08U
X1 = OSD3358_BAS_RefDesignParts_L2:PJ-102B_POWER_CON
X2 = OSD3358_BAS_RefDesignParts_L2:AMP787616-1
X3 = OSD3358_BAS_RefDesignParts_L2:10118192-0001LF: Amphenol FCI Micro USB Type B Complete Surface Mount (SMT) no guide holes
X4 = OSD3358_BAS_RefDesignParts_L2:CTI-JTAG
X5 = OSD3358_BAS_RefDesignParts_L2:SCHA5B0200(ALPS_USD)
X6 = OSD3358_BAS_RefDesignParts_L2:MIKROE_CLICK
Y1 = OSD3358_BAS_RefDesignParts_L2:7A-24.000MAAJ-T
Y2 = OSD3358_BAS_RefDesignParts_L2:ABS07-32.768KHZ-T

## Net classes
0 default: width 0.127 mm, drill 0.254 mm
